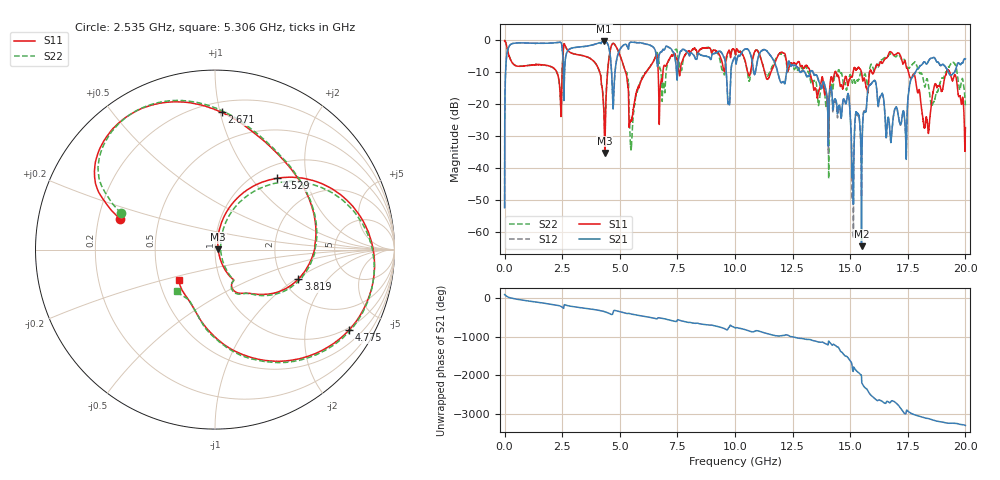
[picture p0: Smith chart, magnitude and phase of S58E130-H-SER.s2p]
!{S58E130}
!Johanson Technology Inc.
!www.johansontechnology.com
!Test Board Conditions:
!Substrate Type  RO4350B
!Substrate Thickness  60 mil
!Substrate Dk  3.66
!TL Type: GCPW
!TL Trace Width  115 mil
!TL Gap  52 mil
!Electrode orientation  Horizontal
!DUT TOPOLOGY	SERIES
!Mounting Pad LxW  55x428 mil
! Created Wed Apr 14 11:05:34 2021
# mhz S ma R 50
! 2 Port Network Data from SP1.SP block
! freq  magS11  angS11  magS21  angS21  magS12  angS12  magS22  angS22
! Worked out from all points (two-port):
!   20001 points, 300 kHz to 20 GHz, reference 50 ohm
!   highest |S21| = -0.29 dB at 4.327 GHz (marker M1); lowest = -64.3 dB at 15.49 GHz (marker M2)
!   |S21| within 3 dB of the highest: 123.9 MHz to 2.509 GHz (2.385 GHz wide, 181 % of centre); 2.734 GHz to 4.556 GHz (1.822 GHz wide, 50 % of centre)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
!   lowest |S11| = -35.2 dB at 4.348 GHz (marker M3), VSWR 1.04, Z = 51.8 + j0.255 ohm
!   |S11| at or under -10 dB: 5.256 GHz to 6.135 GHz (878.8 MHz wide, 15.4 % of centre); 13.26 GHz to 14.33 GHz (1.072 GHz wide, 7.78 % of centre); 17.53 GHz to 19.19 GHz (1.653 GHz wide, 9.01 % of centre)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
!   |S22| runs from -43.2 to 0.0 dB; largest |S21 - S12| = 0.014
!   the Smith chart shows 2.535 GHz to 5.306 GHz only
!   S11 on the Smith chart (normalised r, x): 2.535 GHz: 0.29, +0.15; 2.671 GHz: 0.27, +1.01; 3.819 GHz: 2.41, -1.05; 4.529 GHz: 1.23, +1.35; 4.775 GHz: 0.91, -3.37; 5.306 GHz: 0.64, -0.23
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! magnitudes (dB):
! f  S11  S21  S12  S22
! 300 kHz  -0.1  -52.3  -52.4  -0.1
! 105.3 MHz  -2.3  -4.0  -4.0  -2.3
! 233.3 MHz  -5.6  -1.4  -1.4  -5.6
! 2.535 GHz  -5.1  -5.3  -5.3  -5.0
! 2.671 GHz  -2.3  -4.4  -4.4  -2.3
! 3.334 GHz  -4.7  -2.0  -2.0  -4.6
! 3.819 GHz  -6.2  -1.4  -1.4  -6.2
! 4.327 GHz  -27.0  -0.3  -0.3  -25.8
! 4.348 GHz  -35.2  -0.3  -0.3  -29.9
! 4.529 GHz  -5.6  -2.3  -2.3  -5.5
! 4.775 GHz  -1.2  -11.4  -11.4  -1.2
! 5.306 GHz  -11.6  -1.7  -1.7  -10.1
! 5.509 GHz  -25.0  -0.5  -0.5  -32.5
! 6.667 GHz  -10.0  -6.2  -6.2  -5.3
! 10 GHz  -3.7  -5.1  -5.1  -3.9
! 13.33 GHz  -12.4  -9.4  -9.2  -13.7
! 15.49 GHz  -9.9  -64.3  -46.0  -9.9
! 16.01 GHz  -10.2  -12.7  -12.6  -9.0
! 16.67 GHz  -4.2  -24.3  -24.5  -4.6
! 18.32 GHz  -24.3  -7.4  -7.4  -12.1
! 19.28 GHz  -9.4  -10.1  -10.1  -8.2
! 20 GHz  -27.2  -5.8  -5.7  -20.3
